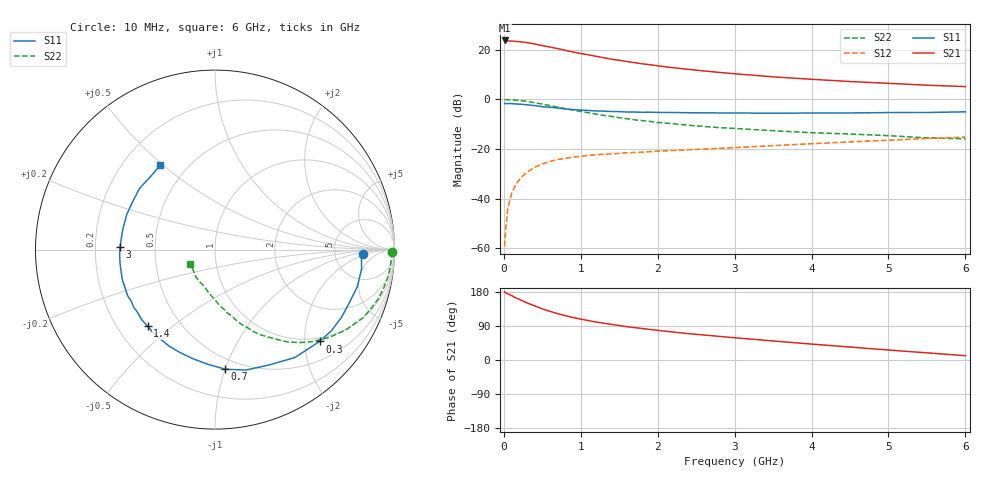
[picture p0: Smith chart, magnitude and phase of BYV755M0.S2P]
! SIEMENS Small Signal Semiconductors
! BFY420
! Si NPN RF SIEGET Grounded Emitter Transistor in MICRO-X
! VCE = 0.75 V  IC = 5 mA
! Common Emitter S-Parameters:  October  1996
# GHz  S  MA  R  50
!  f  S11  S21  S12  S22
! GHz  MAG  ANG  MAG  ANG  MAG  ANG  MAG  ANG
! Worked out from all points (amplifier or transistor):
!   36 points, 10 MHz to 6 GHz, reference 50 ohm
!   highest |S21| = 23.7 dB at 10 MHz (marker M1)
!   |S21| within 3 dB of that: start of sweep to 655.8 MHz
!   unconditionally stable (mu >= 1): 3 GHz to end of sweep
!   at 250 MHz: K = 0.11, MSG = 26.9 dB, |S12| = -30.8 dB
!   at 1.4 GHz: K = 0.56, MSG = 19.1 dB, |S12| = -22.0 dB
!   at 6 GHz: K = 1.17, MAG = 7.7 dB, |S12| = -15.2 dB
!   S11 on the Smith chart (normalised r, x): 10 MHz: 10, -2; 300 MHz: 0.91, -2.35; 700 MHz: 0.41, -1.00; 1.4 GHz: 0.33, -0.41; 3 GHz: 0.31, +0.01; 6 GHz: 0.36, +0.49
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0.01  0.8251 -1.7  15.35 179.9  0.0011 92.4  0.9858 -0.8
0.02  0.8168 -3.1  15.31 177.6  0.0021 89.3  0.9868 -1.6
0.05  0.8238 -7.4  15 174.5  0.0062 87.5  0.983 -4.2
0.1  0.8192 -14.6  14.95 170.3  0.0126 82.4  0.9773 -8.6
0.15  0.8057 -21.0  14.7 164.3  0.0185 77.8  0.9638 -12.8
0.2  0.7997 -28.1  14.5 160.4  0.024 75.1  0.9506 -16.8
0.25  0.7908 -34.8  14.25 155.2  0.029 71.3  0.9288 -20.8
0.3  0.7754 -41.3  13.89 150.7  0.034 68.8  0.9085 -24.7
0.4  0.7481 -53.5  13.04 143.1  0.0426 62.6  0.855 -31.6
0.5  0.7098 -65.0  12.06 134.8  0.05 57.3  0.8014 -37.7
0.6  0.6926 -75.7  11.32 128.4  0.0561 52.9  0.7474 -43.3
0.7  0.6688 -85.1  10.53 122.3  0.0613 48.9  0.6967 -48.1
0.9  0.6213 -100.9  8.974 112.0  0.0685 43.1  0.6055 -55.6
1.1  0.5955 -115.3  7.871 103.9  0.0742 39.1  0.535 -62.2
1.4  0.5684 -131.4  6.434 93.8  0.0793 35.4  0.4522 -69.6
1.7  0.555 -144.7  5.479 85.4  0.0848 33.0  0.3858 -75.5
2.2  0.5431 -161.7  4.33 73.8  0.0931 30.5  0.3228 -83.6
3  0.5298 178.6  3.271 58.7  0.1065 28.7  0.2593 -94.3
3.5  0.5259 168.1  2.839 50.2  0.1167 27.1  0.2335 -100.6
4.5  0.5313 149.5  2.285 34.2  0.1387 22.5  0.2 -114.4
5.5  0.5429 131.2  1.926 18.9  0.1622 16.4  0.167 -136.5
6  0.5604 123.0  1.806 11.3  0.1734 12.8  0.1598 -150.1
